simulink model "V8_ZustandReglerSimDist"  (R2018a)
settings: Solver=ode45  StartTime=0.0  StopTime=10  RelTol=1e-3
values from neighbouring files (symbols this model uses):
  A = [1 1    [V8_1_ZustandRegler.m]    (also in V8_2_ZustandRegler.m; V8_2_ZustandRegler_dist.m; V8_3_ZustandRegler.m = [-1, 0, 0; V8_5_ZustandRegler.m)
  B = [0; 1]    [V8_1_ZustandRegler.m]    (also in V8_2_ZustandRegler.m; V8_2_ZustandRegler_dist.m; V8_3_ZustandRegler.m = [1; 0; 0]; V8_5_ZustandRegler.m)
  C = [1 0]    [V8_1_ZustandRegler.m]    (also in V8_2_ZustandRegler.m; V8_2_ZustandRegler_dist.m; V8_5_ZustandRegler.m; V8_7_ZustandRegler.m)
  F = place(A,B,pd)    [V8_1_ZustandRegler.m]    (also in V8_2_ZustandRegler.m; V8_2_ZustandRegler_dist.m; V8_3_ZustandRegler.m = S_c_n' * PA; V8_5_ZustandRegler.m)
  G = place(Ae,Be,pde)    [V8_2_ZustandRegler_dist.m]
  V = inv(C*inv(B*F-A)*B)    [V8_2_ZustandRegler.m]    (also in V8_2_ZustandRegler_dist.m)

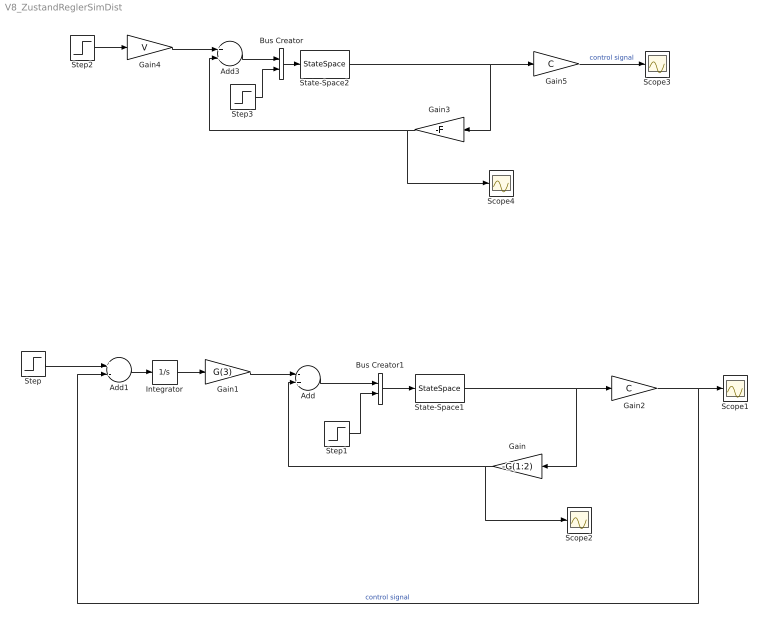
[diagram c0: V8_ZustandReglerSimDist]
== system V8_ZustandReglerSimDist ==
  Add : Sum  Inputs=-+
  Add1 : Sum  Inputs=+-
  Add3 : Sum
  Bus Creator : BusCreator  Inputs=2
  Bus Creator1 : BusCreator  Inputs=2
  Gain : Gain  Gain=-G(1:2)  Multiplication=Matrix(K*u)
  Gain1 : Gain  Gain=G(3)
  Gain2 : Gain  Gain=C  Multiplication=Matrix(K*u)
  Gain3 : Gain  Gain=-F  Multiplication=Matrix(K*u)
  Gain4 : Gain  Gain=V
  Gain5 : Gain  Gain=C  Multiplication=Matrix(K*u)
  Integrator : Integrator
  Scope{1..4} (4 alike) : Scope
  State-Space1 : StateSpace  A=A  B=[B B]  C=eye(2)  D=zeros(2,2)  InitialCondition=[2; 2]
  State-Space2 : StateSpace  A=A  B=[B B]  C=eye(2)  D=zeros(2,2)  InitialCondition=[2; 2]
  Step : Step  Time=0  SampleTime=0
  Step1 : Step  Time=2  After=10  SampleTime=0
  Step2 : Step  Time=0  SampleTime=0
  Step3 : Step  Time=2  After=10  SampleTime=0
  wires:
  Gain/1 -> Add/2, Scope2/1
  Gain2/1 -> Add1/2, Scope1/1  "control signal"
  Integrator/1 -> Gain1/1
  Add1/1 -> Integrator/1
  Step/1 -> Add1/1
  Gain1/1 -> Add/1
  State-Space1/1 -> Gain/1, Gain2/1
  Gain5/1 -> Scope3/1  "control signal"
  Gain4/1 -> Add3/1
  Step2/1 -> Gain4/1
  State-Space2/1 -> Gain3/1, Gain5/1
  Gain3/1 -> Add3/2, Scope4/1
  Add3/1 -> Bus Creator/1
  Bus Creator/1 -> State-Space2/1
  Step3/1 -> Bus Creator/2
  Add/1 -> Bus Creator1/1
  Step1/1 -> Bus Creator1/2
  Bus Creator1/1 -> State-Space1/1
